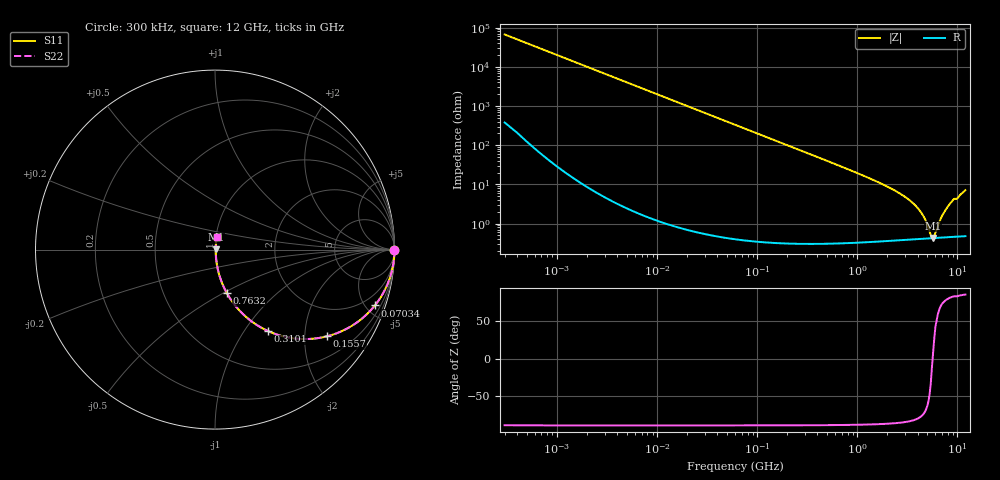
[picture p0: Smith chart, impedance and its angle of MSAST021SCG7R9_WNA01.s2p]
! MSAST021SCG7R9_WNA01  S-PARAMETER MODEL  ( General Type )
! Model Generated by TAIYO YUDEN Corporation (http://www.ty-top.com)
! Version 2.0
! TAIYO YUDEN Control No. 181101
! Copyright(c) 2015 TAIYO YUDEN CO.,LTD. All Rights Reserved.
! Product Description (link to TY-COMPAS)
! https://ds.yuden.co.jp/TYCOMPAS/or/detail?pn=MSAST021SCG7R9CWNA01&u=M
! Products Name : Multilayer Ceramic Capacitors
! Characteristics :
!  Capacitance : 7.9 pF , Rated Voltage : 25V , TCC : CG / C0G
!  Case Size : 0.25 x 0.125 / 0.0098 x 0.0049 [mm/inch] , Thickness : 0.125 / 0.0049 [mm/inch]
!  (Conditions: Temperature = 25 degC , DC Bias Current/Voltage = 0A / 0V)
! External Node Assignments :
!  1  o---| |---o  2
! GND o---------o GND
! Frequency Range : 0.3MHz  -  12000MHz  [ 401 STEP ]
# MHz S RI R 50
! Freq[MHz].  S11 Real  S11 Imag  S21 Real  S21 Imag  S12 Real  S12 Imag  S22 Real  S22 Imag
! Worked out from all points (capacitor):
!   401 points, 300 kHz to 12 GHz, reference 50 ohm
!   read as one part in series: C = 7.9 pF near 316.3 kHz
!   lowest |Z| = 435 mohm at 5.715 GHz (marker M1)
!   series resonance near 5.646 GHz, so ESL is about 100 pH
!   S11 on the Smith chart (normalised r, x): 300 kHz: open; 70.34 MHz: 1.01, -5.73; 155.7 MHz: 1.01, -2.59; 310.1 MHz: 1.01, -1.30; 763.2 MHz: 1.01, -0.52; 12 GHz: 1.01, +0.14
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0.3  1 -0.00149  1.07e-05 0.00149  1.07e-05 0.00149  1 -0.00149
1.769972  0.9999 -0.00878  8.53e-05 0.00878  8.53e-05 0.00878  0.9999 -0.00878
10.44266  0.9973 -0.0517  0.00271 0.0517  0.00271 0.0517  0.9973 -0.0517
27.10171  0.9821 -0.1321  0.0179 0.1321  0.0179 0.1321  0.9821 -0.1321
60  0.9182 -0.2734  0.0818 0.2734  0.0818 0.2734  0.9182 -0.2734
70.33673  0.891 -0.311  0.109 0.311  0.109 0.311  0.891 -0.311
104.6549  0.787 -0.4086  0.213 0.4086  0.213 0.4086  0.787 -0.4086
155.7172  0.6253 -0.4828  0.3747 0.4828  0.3747 0.4828  0.6253 -0.4828
310.0777  0.2964 -0.4543  0.7036 0.4543  0.7036 0.4543  0.2964 -0.4543
353.9943  0.2444 -0.427  0.7556 0.427  0.7556 0.427  0.2444 -0.427
763.2128  0.0655 -0.2414  0.9345 0.2414  0.9345 0.2414  0.0655 -0.2414
2088.533  0.0104 -0.082  0.9896 0.082  0.9896 0.082  0.0104 -0.082
3026.31  0.00606 -0.0469  0.9939 0.0469  0.9939 0.0469  0.00606 -0.0469
3944.255  0.00469 -0.0258  0.9953 0.0258  0.9953 0.0258  0.00469 -0.0258
4623.766  0.00433 -0.014  0.9957 0.014  0.9957 0.014  0.00433 -0.014
5420.343  0.00425 -0.00267  0.9958 0.00267  0.9958 0.00267  0.00425 -0.00267
5715.274  0.00428 0.00068  0.9957 -0.00068  0.9957 -0.00068  0.00428 0.00068
6026.253  0.00433 0.00401  0.9957 -0.00401  0.9957 -0.00401  0.00433 0.00401
7064.448  0.00466 0.0155  0.9953 -0.0155  0.9953 -0.0155  0.00466 0.0155
8064.993  0.00524 0.027  0.9948 -0.027  0.9948 -0.027  0.00524 0.027
8966.534  0.00608 0.0385  0.9939 -0.0385  0.9939 -0.0385  0.00608 0.0385
12000  0.0098 0.0705  0.9902 -0.0705  0.9902 -0.0705  0.0098 0.0705
